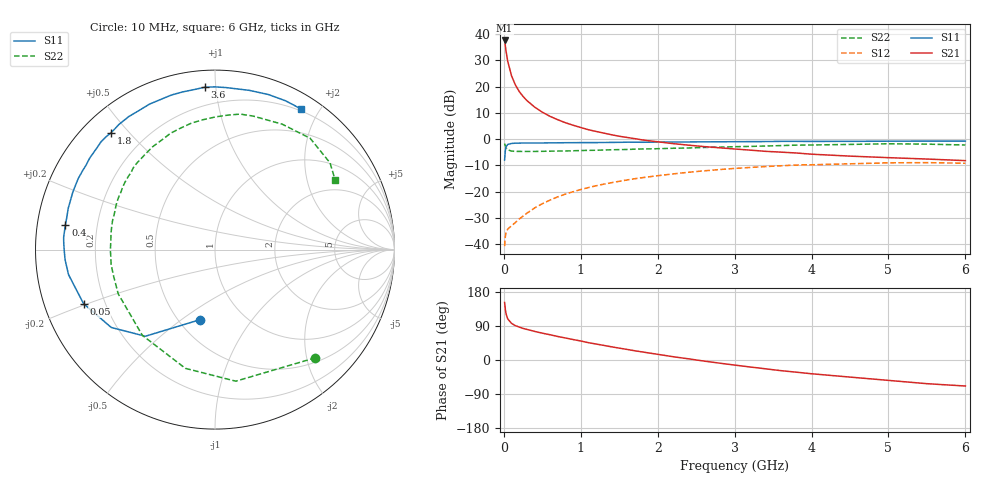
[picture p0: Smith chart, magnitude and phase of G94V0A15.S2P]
! SIEMENS Small Signal Semiconductors
! BFG235
! Si NPN RF Bipolar Junction Transistor in SOT223
! VCE = 4 V  IC = 150 mA
! Common Emitter S-Parameters:  July  1994
# GHz  S  MA  R  50
!  f  S11  S21  S12  S22
! GHz  MAG  ANG  MAG  ANG  MAG  ANG  MAG  ANG
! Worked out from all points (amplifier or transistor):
!   40 points, 10 MHz to 6 GHz, reference 50 ohm
!   highest |S21| = 37.5 dB at 10 MHz (marker M1)
!   |S21| within 3 dB of that: start of sweep to 23.93 MHz
!   unconditionally stable (mu >= 1): 448.8 MHz to 1.506 GHz
!   at 200 MHz: K = 0.81, MSG = 24.3 dB, |S12| = -30.4 dB
!   at 1.5 GHz: K = 1.00, MAG = 8.4 dB, |S12| = -16.0 dB
!   at 6 GHz: K = 0.90, MSG = 0.5 dB, |S12| = -9.2 dB
!   S11 on the Smith chart (normalised r, x): 10 MHz: 0.63, -0.59; 50 MHz: 0.12, -0.20; 400 MHz: 0.08, +0.08; 1.8 GHz: 0.08, +0.44; 3.6 GHz: 0.09, +0.93; 6 GHz: 0.18, +1.77
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0.01  0.4002 -102.3  75.32 151.9  0.0092 62.8  0.8225 -47.1
0.02  0.6194 -128.8  58.75 132.8  0.0142 48.0  0.7423 -81.0
0.03  0.7227 -143.1  45.9 121.0  0.0169 40.8  0.6819 -104.0
0.05  0.7918 -157.6  30.41 108.6  0.0194 34.3  0.626 -130.3
0.1  0.8279 -170.3  16.02 96.7  0.0225 37.3  0.5929 -155.5
0.15  0.8373 -176.2  10.75 90.7  0.0259 43.9  0.5839 -166.1
0.2  0.8399 -179.6  8.045 86.9  0.0302 48.4  0.5845 -171.9
0.25  0.8434 177.6  6.484 83.4  0.0343 51.9  0.5819 -176.1
0.3  0.8461 175.4  5.412 80.8  0.039 54.5  0.5829 -179.6
0.4  0.8449 170.7  4.072 75.5  0.049 57.2  0.5824 175.4
0.5  0.8453 167.4  3.255 70.8  0.0591 58.5  0.5862 171.2
0.6  0.8495 164.3  2.714 66.7  0.0692 58.2  0.5899 167.4
0.7  0.8511 160.6  2.343 62.1  0.0797 57.7  0.5935 163.9
0.9  0.8559 155.2  1.839 54.0  0.0996 54.8  0.6003 157.6
1.1  0.8587 148.9  1.509 45.7  0.1198 51.3  0.6113 151.4
1.8  0.8714 131.8  0.967 21.3  0.1847 36.6  0.6497 132.0
2.2  0.8832 123.0  0.821 8.7  0.2178 27.6  0.67 121.3
3.2  0.8968 101.6  0.618 -18.4  0.289 4.4  0.7267 95.3
3.6  0.9065 93.6  0.566 -28.1  0.3109 -5.5  0.7532 84.4
4.5  0.9076 77.8  0.475 -45.1  0.3392 -25.2  0.7927 61.9
5.5  0.9176 64.6  0.418 -62.5  0.3572 -46.9  0.8027 37.0
6  0.9185 58.7  0.39 -68.7  0.3476 -55.1  0.7731 30.0
